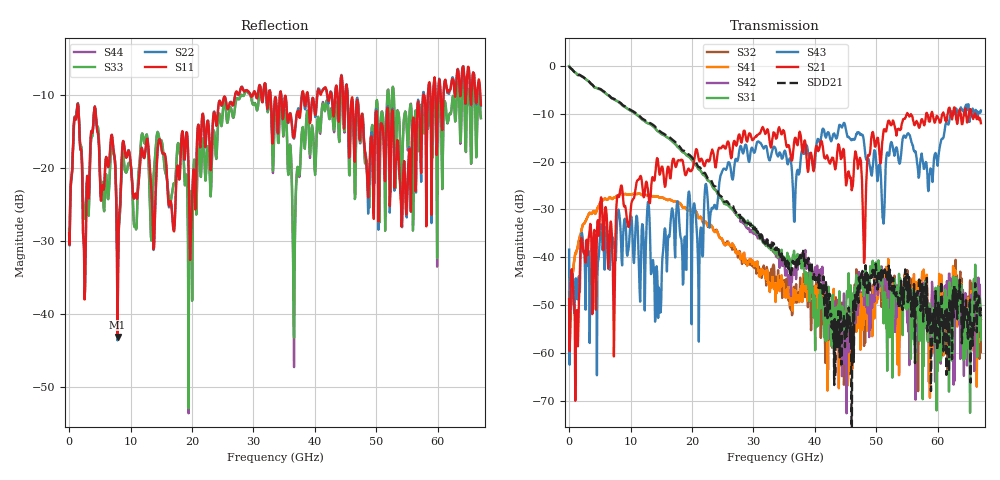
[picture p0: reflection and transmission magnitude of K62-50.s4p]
!Agilent Technologies,N5247A,US50470101,A.10.25.02
!Agilent N5247A: A.10.25.02
!Date: Tuesday, May 12, 2015 13:43:05
!Correction: Sdd11(Full 4 Port(1,2,3,4))
!Sdc11(Full 4 Port(1,2,3,4))
!Sdd12(Full 4 Port(1,2,3,4))
!Sdc12(Full 4 Port(1,2,3,4))
!Scd11(Full 4 Port(1,2,3,4))
!Scc11(Full 4 Port(1,2,3,4))
!Scd12(Full 4 Port(1,2,3,4))
!Scc12(Full 4 Port(1,2,3,4))
!Sdd21(Full 4 Port(1,2,3,4))
!Sdc21(Full 4 Port(1,2,3,4))
!Sdd22(Full 4 Port(1,2,3,4))
!Sdc22(Full 4 Port(1,2,3,4))
!Scd21(Full 4 Port(1,2,3,4))
!Scc21(Full 4 Port(1,2,3,4))
!Scd22(Full 4 Port(1,2,3,4))
!Scc22(Full 4 Port(1,2,3,4))
!Balanced Topology: BBAL
!S4P File: Measurements: <Sdd11,Sdc11,Sdd12,Sdc12>,
!<Scd11,Scc11,Scd12,Scc12>,
!<Sdd21,Sdc21,Sdd22,Sdc22>,
!<Scd21,Scc21,Scd22,Scc22>:
# Hz S  dB  R 50
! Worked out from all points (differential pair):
!   801 points, 10 MHz to 67 GHz, reference 50 ohm
!   strongest paths, dB at 10 MHz, 16.76 GHz, 33.51 GHz, 50.25 GHz, 67 GHz:
!     S21: -48.8, -20.4, -14.3, -15.1, -12.0
!     S43: -38.4, -29.8, -17.1, -23.3, -9.3
!     S31: -0.1, -15.7, -39.3, -44.6, -57.3
!     S42: -0.1, -15.7, -38.8, -48.0, -52.6
!     S41: -47.2, -28.2, -45.8, -48.7, -53.1
!     S32: -50.7, -28.2, -44.9, -47.6, -51.6
!   taken as a pair (ports 1,2 in; 3,4 out), SDD21 dB: 0.0, -15.4, -38.4, -45.9, -52.3
!   lowest |S11| = -43.1 dB at 7.881 GHz (marker M1), VSWR 1.01, Z = 50.1 - j0.696 ohm
!   |S11| at or under -10 dB: start of sweep to 27 GHz; 34.52 GHz to 37.89 GHz (3.368 GHz wide, 9.3 % of centre); 45.31 GHz to 57.64 GHz (12.33 GHz wide, 23.9 % of centre)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
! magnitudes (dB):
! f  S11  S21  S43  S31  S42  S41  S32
! 10 MHz  -28.9  -48.8  -38.4  -0.1  -0.1  -47.2  -50.7
! 7.881 GHz  -43.1  -27.2  -31.0  -7.4  -7.4  -27.2  -27.2
! 14.75 GHz  -16.0  -22.8  -49.4  -13.9  -13.9  -27.6  -27.5
! 27.89 GHz  -9.1  -15.3  -16.7  -31.8  -32.6  -40.5  -40.1
! 36.6 GHz  -15.8  -16.0  -32.5  -38.6  -43.7  -49.5  -46.2
! 45.14 GHz  -8.5  -24.6  -14.1  -48.1  -72.6  -56.7  -51.3
! 67 GHz  -11.3  -12.0  -9.3  -57.3  -52.6  -53.1  -51.6
